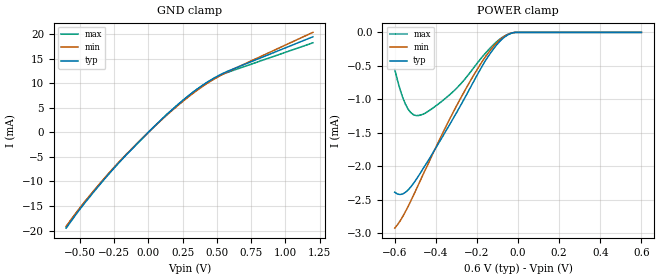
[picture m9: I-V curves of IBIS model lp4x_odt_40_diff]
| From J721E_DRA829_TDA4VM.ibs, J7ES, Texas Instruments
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|   Model lp4x_odt_40_diff
[Model] lp4x_odt_40_diff
Model_type Input
Polarity   Non-Inverting
Enable   Active-High
Vinl =  0.0V
Vinh =  0.900V
C_comp   1.900pF   1.700pF   2.112pF
[Model Spec]
Vinh   0.900V   0.900V   0.900V
Vinl   0.0V   0.0V   0.0V
[Temperature Range]   25.000   0.125k   -40.000
[Voltage Range]   0.600V   0.570V   0.650V
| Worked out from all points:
|   GND clamp passes 1 mA (typ) near -0.04 V on its own axis
|   POWER clamp passes 1 mA (typ) near -0.26 V on its own axis
[GND_clamp]
|Voltage   I(typ)   I(min)   I(max)
-600mV    -19.51mA   -19.12mA   -19.31mA
-457mV    -14.13mA   -13.87mA   -13.89mA
-300mV    -8.872mA   -8.686mA   -8.742mA
-170mV    -4.857mA   -4.729mA   -4.807mA
117mV     3.175mA    3.06mA     3.161mA
235mV     6.109mA    5.908mA    6.086mA
339mV     8.442mA    8.198mA    8.408mA
443mV     10.44mA    10.21mA    10.37mA
561mV     12.21mA    12.07mA    12.01mA
1.2V      19.43mA    20.33mA    18.2mA
[POWER_clamp]
|Voltage   I(typ)   I(min)   I(max)
-600mV    -2.386mA   -2.922mA   -552uA
-561mV    -2.412mA   -2.749mA   -972.7uA
-535mV    -2.352mA   -2.599mA   -1.146mA
-509mV    -2.255mA   -2.433mA   -1.229mA
-470mV    -2.074mA   -2.174mA   -1.23mA
-339mV    -1.409mA   -1.333mA   -947.8uA
-235mV    -841.7uA   -739.8uA   -606uA
-157mV    -413uA     -355.4uA   -306.1uA
-78.26mV  -102.7uA   -85.16uA   -78.05uA
-39.13mV  -21.14uA   -17.01uA   -16.53uA
-13.04mV  0A         0A         0A
600mV     0A         0A         0A
